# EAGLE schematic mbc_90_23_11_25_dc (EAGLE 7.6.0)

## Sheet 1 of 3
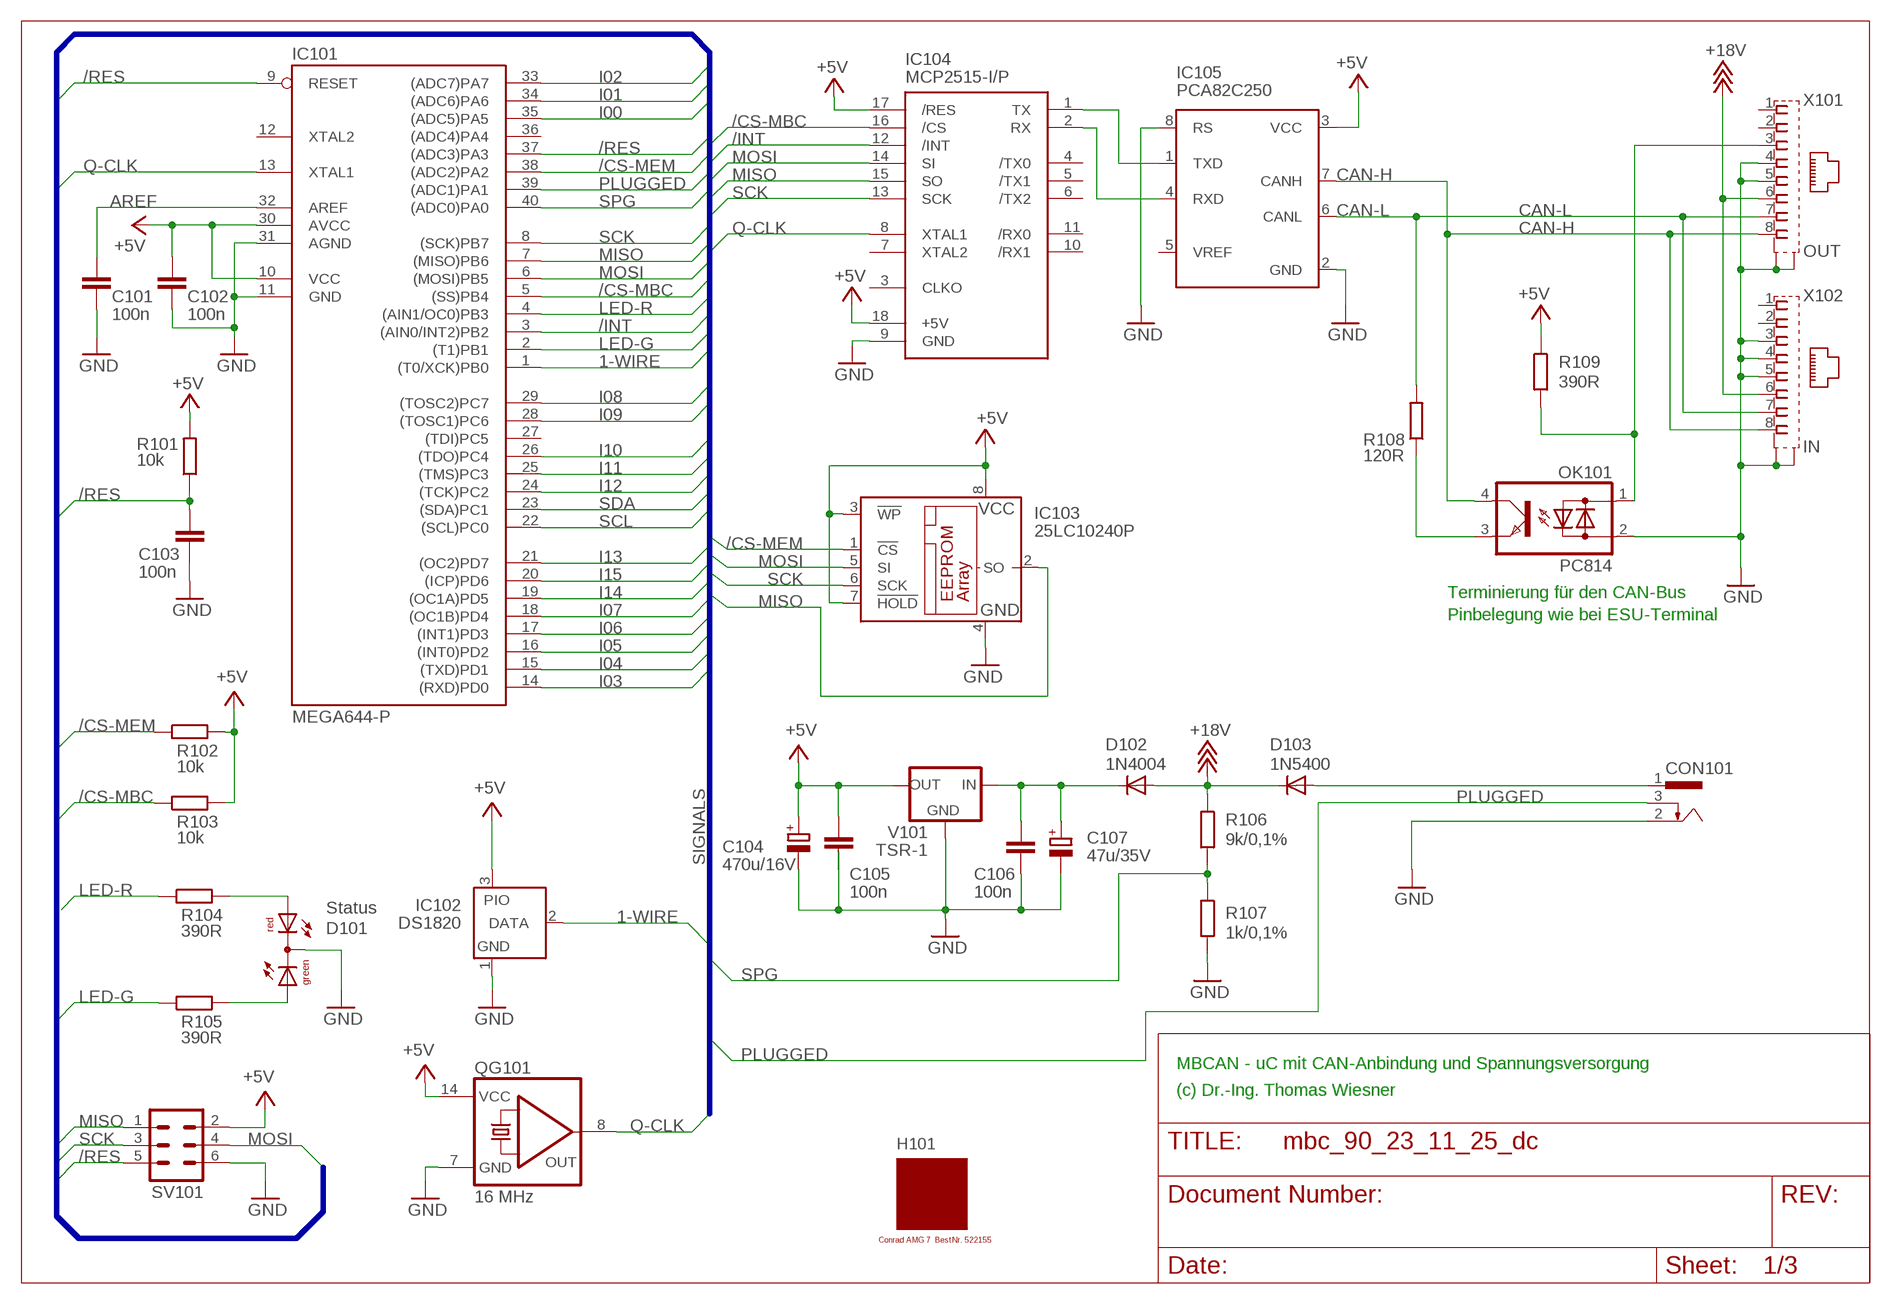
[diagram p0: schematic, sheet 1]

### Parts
C101  100n  C-EU025-025X050  [C025-025X050]
C102  100n  C-EU025-025X050  [C025-025X050]
C103  100n  C-EU025-025X050  [C025-025X050]
C104  470u/16V  CPOL-EUE3.5-8  [E3,5-8]
C105  100n  C-EU025-025X050  [C025-025X050]
C106  100n  C-EU025-025X050  [C025-025X050]
C107  47u/35V  CPOL-EUE2.5-7  [E2,5-7]
CON101  POWER-JACK  [POWER-JACK]
D101  Status  DUOLED5MM  [DUOLED5MM]
D102  1N4004  [DO41-10]
D103  1N5400  [DO201-15]
H101  MODULGEHÄUSE-AMG-7  [MODULGEHÄUSE-1]
IC101  MEGA644-P  MEGA323-P  [DIL40]
IC102  DS1820  DS2405  [TO92-]
IC103  25LC10240P  25LC040P  [DIL8]
IC104  MCP2515-I/P  MCP2510-I/P  [DIL18]
IC105  PCA82C250  [DIL08]
OK101  PC814  [DIL04]
QG101  16 MHz  QG5860  [DIL14S]
R101  10k  R-EU_0207/10  [0207/10]
R102  10k  R-EU_0207/10  [0207/10]
R103  10k  R-EU_0207/10  [0207/10]
R104  390R  R-EU_0207/10  [0207/10]
R105  390R  R-EU_0207/10  [0207/10]
R106  9k/0,1%  R-EU_0207/10  [0207/10]
R107  1k/0,1%  R-EU_0207/10  [0207/10]
R108  120R  R-EU_0207/10  [0207/10]
R109  390R  R-EU_0207/10  [0207/10]
SV101  ML6  [ML6]
V101  TSR-1  [TRACO-TSR-1]
X101  OUT  0446200002  [0446200002]
X102  IN  0446200002  [0446200002]

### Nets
1-WIRE: IC101.1((T0/XCK)PB0) IC102.2(DATA)
+5V: C102.1 C104.+ C105.1 IC101.10(VCC) IC101.30(AVCC) IC102.3(PIO) IC103.3(!WP) IC103.7(!HOLD) IC103.8(VCC) IC104.17(/RES) IC104.18(+5V) IC105.3(VCC) QG101.14(VCC) R101.2 R102.2 R103.2 R109.1 SV101.2 V101.OUT ; also sheet 2
+18V: D102.A D103.C R106.1 X101.6 X102.6
/CS-MBC: IC101.5((SS)PB4) IC104.16(/CS) R103.1
/CS-MEM: IC101.38((ADC2)PA2) IC103.1(!CS) R102.1
/INT: IC101.3((AIN0/INT2)PB2) IC104.12(/INT)
/RES: C103.1 IC101.9(RESET) IC101.37((ADC3)PA3) R101.1 SV101.5
AREF: C101.1 IC101.32(AREF)
CAN-H: IC105.7(CANH) OK101.4(C) X101.8 X102.8
CAN-L: IC105.6(CANL) R108.2 X101.7 X102.7
GND: C101.2 C102.2 C103.2 C104.- C105.2 C106.2 C107.- CON101.2 D101.K(C) IC101.11(GND) IC101.31(AGND) IC102.1(GND) IC103.4(GND) IC104.9(GND) IC105.2(GND) IC105.8(RS) QG101.7(GND) R107.2 SV101.6 V101.GND X101.4 X101.5 X101.S@1(S1) X101.S@2(S2) X102.3 X102.4 X102.5 X102.S@1(S1) X102.S@2(S2) ; also sheet 2
I00: IC101.35((ADC5)PA5) ; also sheet 2
I01: IC101.34((ADC6)PA6) ; also sheet 2
I02: IC101.33((ADC7)PA7) ; also sheet 2
I03: IC101.14((RXD)PD0) ; also sheet 2
I04: IC101.15((TXD)PD1) ; also sheet 2
I05: IC101.16((INT0)PD2) ; also sheet 2
I06: IC101.17((INT1)PD3) ; also sheet 2
I07: IC101.18((OC1B)PD4) ; also sheet 2
I08: IC101.29((TOSC2)PC7) ; also sheet 2
I09: IC101.28((TOSC1)PC6) ; also sheet 2
I10: IC101.26((TDO)PC4) ; also sheet 2
I11: IC101.25((TMS)PC3) ; also sheet 2
I12: IC101.24((TCK)PC2) ; also sheet 2
I13: IC101.21((OC2)PD7) ; also sheet 2
I14: IC101.19((OC1A)PD5) ; also sheet 2
I15: IC101.20((ICP)PD6) ; also sheet 2
LED-G: IC101.2((T1)PB1) R105.1
LED-R: IC101.4((AIN1/OC0)PB3) R104.1
MISO: IC101.7((MISO)PB6) IC103.2(SO) IC104.15(SO) SV101.1
MOSI: IC101.6((MOSI)PB5) IC103.5(SI) IC104.14(SI) SV101.4
N$1: IC104.1(TX) IC105.1(TXD)
N$2: IC104.2(RX) IC105.4(RXD)
N$4: OK101.3(E) R108.1
N$6: C106.1 C107.+ D102.C V101.IN
N$7: OK101.1(AC1) R109.2 X101.3
N$9: D101.AR R104.2
N$13: D101.AG R105.2
PLUGGED: CON101.3 IC101.39((ADC1)PA1)
Q-CLK: IC101.13(XTAL1) IC104.8(XTAL1) QG101.8(OUT)
SCK: IC101.8((SCK)PB7) IC103.6(SCK) IC104.13(SCK) SV101.3
SCL: IC101.22((SCL)PC0) ; also sheet 2
SDA: IC101.23((SDA)PC1) ; also sheet 2
SPG: IC101.40((ADC0)PA0) R106.2 R107.1
V-NETZTEIL1: CON101.1 D103.A
Unconnected: IC101.12(XTAL2) IC101.27((TDI)PC5) IC101.36((ADC4)PA4) IC104.3(CLKO) IC104.4(/TX0) IC104.5(/TX1) IC104.6(/TX2) IC104.7(XTAL2) IC104.10(/RX1) IC104.11(/RX0) IC105.5(VREF) OK101.2(AC2) X101.1 X101.2 X102.1 X102.2

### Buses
SIGNALS

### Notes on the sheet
- Terminierung für den CAN-Bus
- Pinbelegung wie bei ESU-Terminal
- MBCAN - uC mit CAN-Anbindung und Spannungsversorgung
- (c) Dr.-Ing. Thomas Wiesner

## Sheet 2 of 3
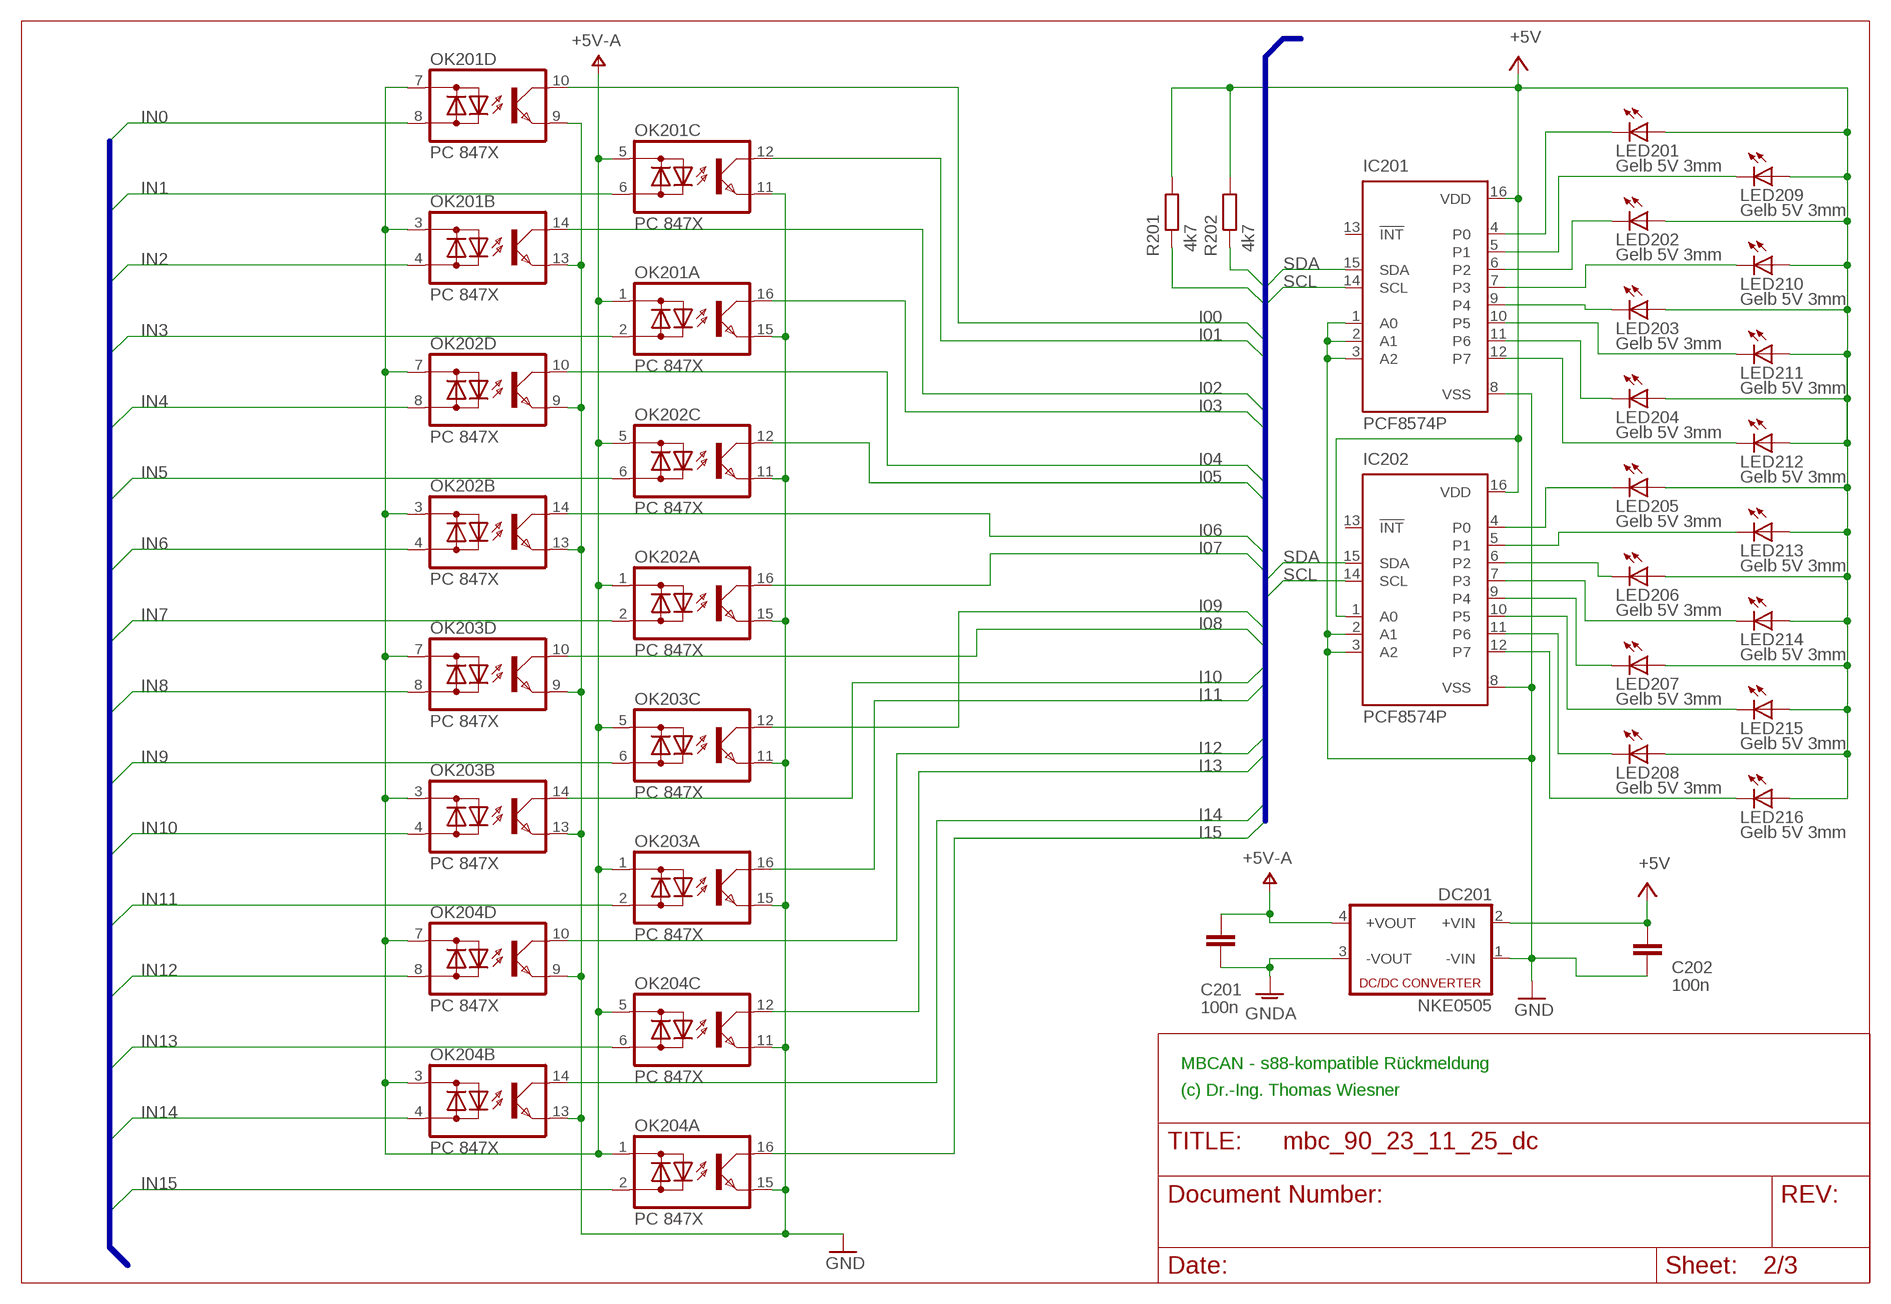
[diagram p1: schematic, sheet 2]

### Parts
C201  100n  C-EU025-025X050  [C025-025X050]
C202  100n  C-EU025-025X050  [C025-025X050]
DC201  NKE0505  NME  [NME]
IC201  PCF8574P  [DIL16]
IC202  PCF8574P  [DIL16]
LED201  Gelb 5V 3mm  LED3MM  [LED3MM]
LED202  Gelb 5V 3mm  LED3MM  [LED3MM]
LED203  Gelb 5V 3mm  LED3MM  [LED3MM]
LED204  Gelb 5V 3mm  LED3MM  [LED3MM]
LED205  Gelb 5V 3mm  LED3MM  [LED3MM]
LED206  Gelb 5V 3mm  LED3MM  [LED3MM]
LED207  Gelb 5V 3mm  LED3MM  [LED3MM]
LED208  Gelb 5V 3mm  LED3MM  [LED3MM]
LED209  Gelb 5V 3mm  LED3MM  [LED3MM]
LED210  Gelb 5V 3mm  LED3MM  [LED3MM]
LED211  Gelb 5V 3mm  LED3MM  [LED3MM]
LED212  Gelb 5V 3mm  LED3MM  [LED3MM]
LED213  Gelb 5V 3mm  LED3MM  [LED3MM]
LED214  Gelb 5V 3mm  LED3MM  [LED3MM]
LED215  Gelb 5V 3mm  LED3MM  [LED3MM]
LED216  Gelb 5V 3mm  LED3MM  [LED3MM]
OK201  PC 847X  TIL196  [DIL16]
OK202  PC 847X  TIL196  [DIL16]
OK203  PC 847X  TIL196  [DIL16]
OK204  PC 847X  TIL196  [DIL16]
R201  4k7  R-EU_0207/10  [0207/10]
R202  4k7  R-EU_0207/10  [0207/10]

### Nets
+5V: C202.1 DC201.2(+VIN) IC201.16(VDD) IC202.1(A0) IC202.16(VDD) LED201.A LED202.A LED203.A LED204.A LED205.A LED206.A LED207.A LED208.A LED209.A LED210.A LED211.A LED212.A LED213.A LED214.A LED215.A LED216.A R201.2 R202.2 ; also sheet 1
GND: C202.2 DC201.1(-VIN) IC201.1(A0) IC201.2(A1) IC201.3(A2) IC201.8(VSS) IC202.2(A1) IC202.3(A2) IC202.8(VSS) OK201.9(D:E) OK201.11(C:E) OK201.13(B:E) OK201.15(A:E) OK202.9(D:E) OK202.11(C:E) OK202.13(B:E) OK202.15(A:E) OK203.9(D:E) OK203.11(C:E) OK203.13(B:E) OK203.15(A:E) OK204.9(D:E) OK204.11(C:E) OK204.13(B:E) OK204.15(A:E) ; also sheet 1
GNDA: C201.2 DC201.3(-VOUT) ; also sheet 3
I00: OK201.10(D:C) ; also sheet 1
I01: OK201.12(C:C) ; also sheet 1
I02: OK201.14(B:C) ; also sheet 1
I03: OK201.16(A:C) ; also sheet 1
I04: OK202.10(D:C) ; also sheet 1
I05: OK202.12(C:C) ; also sheet 1
I06: OK202.14(B:C) ; also sheet 1
I07: OK202.16(A:C) ; also sheet 1
I08: OK203.10(D:C) ; also sheet 1
I09: OK203.12(C:C) ; also sheet 1
I10: OK203.14(B:C) ; also sheet 1
I11: OK203.16(A:C) ; also sheet 1
I12: OK204.10(D:C) ; also sheet 1
I13: OK204.12(C:C) ; also sheet 1
I14: OK204.14(B:C) ; also sheet 1
I15: OK204.16(A:C) ; also sheet 1
IN0: OK201.8(D:AC2) ; also sheet 3
IN1: OK201.6(C:AC2) ; also sheet 3
IN2: OK201.4(B:AC2) ; also sheet 3
IN3: OK201.2(A:AC2) ; also sheet 3
IN4: OK202.8(D:AC2) ; also sheet 3
IN5: OK202.6(C:AC2) ; also sheet 3
IN6: OK202.4(B:AC2) ; also sheet 3
IN7: OK202.2(A:AC2) ; also sheet 3
IN8: OK203.8(D:AC2) ; also sheet 3
IN9: OK203.6(C:AC2) ; also sheet 3
IN10: OK203.4(B:AC2) ; also sheet 3
IN11: OK203.2(A:AC2) ; also sheet 3
IN12: OK204.8(D:AC2) ; also sheet 3
IN13: OK204.6(C:AC2) ; also sheet 3
IN14: OK204.4(B:AC2) ; also sheet 3
IN15: OK204.2(A:AC2) ; also sheet 3
N$15: IC201.9(P4) LED203.K(C)
N$31: IC201.10(P5) LED211.K(C)
N$49: IC202.4(P0) LED205.K(C)
N$50: IC201.4(P0) LED201.K(C)
N$51: IC201.5(P1) LED209.K(C)
N$52: IC201.6(P2) LED202.K(C)
N$53: IC201.7(P3) LED210.K(C)
N$54: IC201.11(P6) LED204.K(C)
N$55: IC201.12(P7) LED212.K(C)
N$56: IC202.9(P4) LED207.K(C)
N$57: IC202.5(P1) LED213.K(C)
N$58: IC202.6(P2) LED206.K(C)
N$59: IC202.7(P3) LED214.K(C)
N$60: IC202.10(P5) LED215.K(C)
N$61: IC202.11(P6) LED208.K(C)
N$62: IC202.12(P7) LED216.K(C)
SCL: IC201.14(SCL) IC202.14(SCL) R201.1 ; also sheet 1
SDA: IC201.15(SDA) IC202.15(SDA) R202.1 ; also sheet 1
V+: C201.1 DC201.4(+VOUT) OK201.1(A:AC1) OK201.3(B:AC1) OK201.5(C:AC1) OK201.7(D:AC1) OK202.1(A:AC1) OK202.3(B:AC1) OK202.5(C:AC1) OK202.7(D:AC1) OK203.1(A:AC1) OK203.3(B:AC1) OK203.5(C:AC1) OK203.7(D:AC1) OK204.1(A:AC1) OK204.3(B:AC1) OK204.5(C:AC1) OK204.7(D:AC1) ; supply symbol labelled +5V-A
Unconnected: IC201.13(!INT) IC202.13(!INT)

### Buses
B$1
B$2

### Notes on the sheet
- MBCAN - s88-kompatible Rückmeldung
- (c) Dr.-Ing. Thomas Wiesner

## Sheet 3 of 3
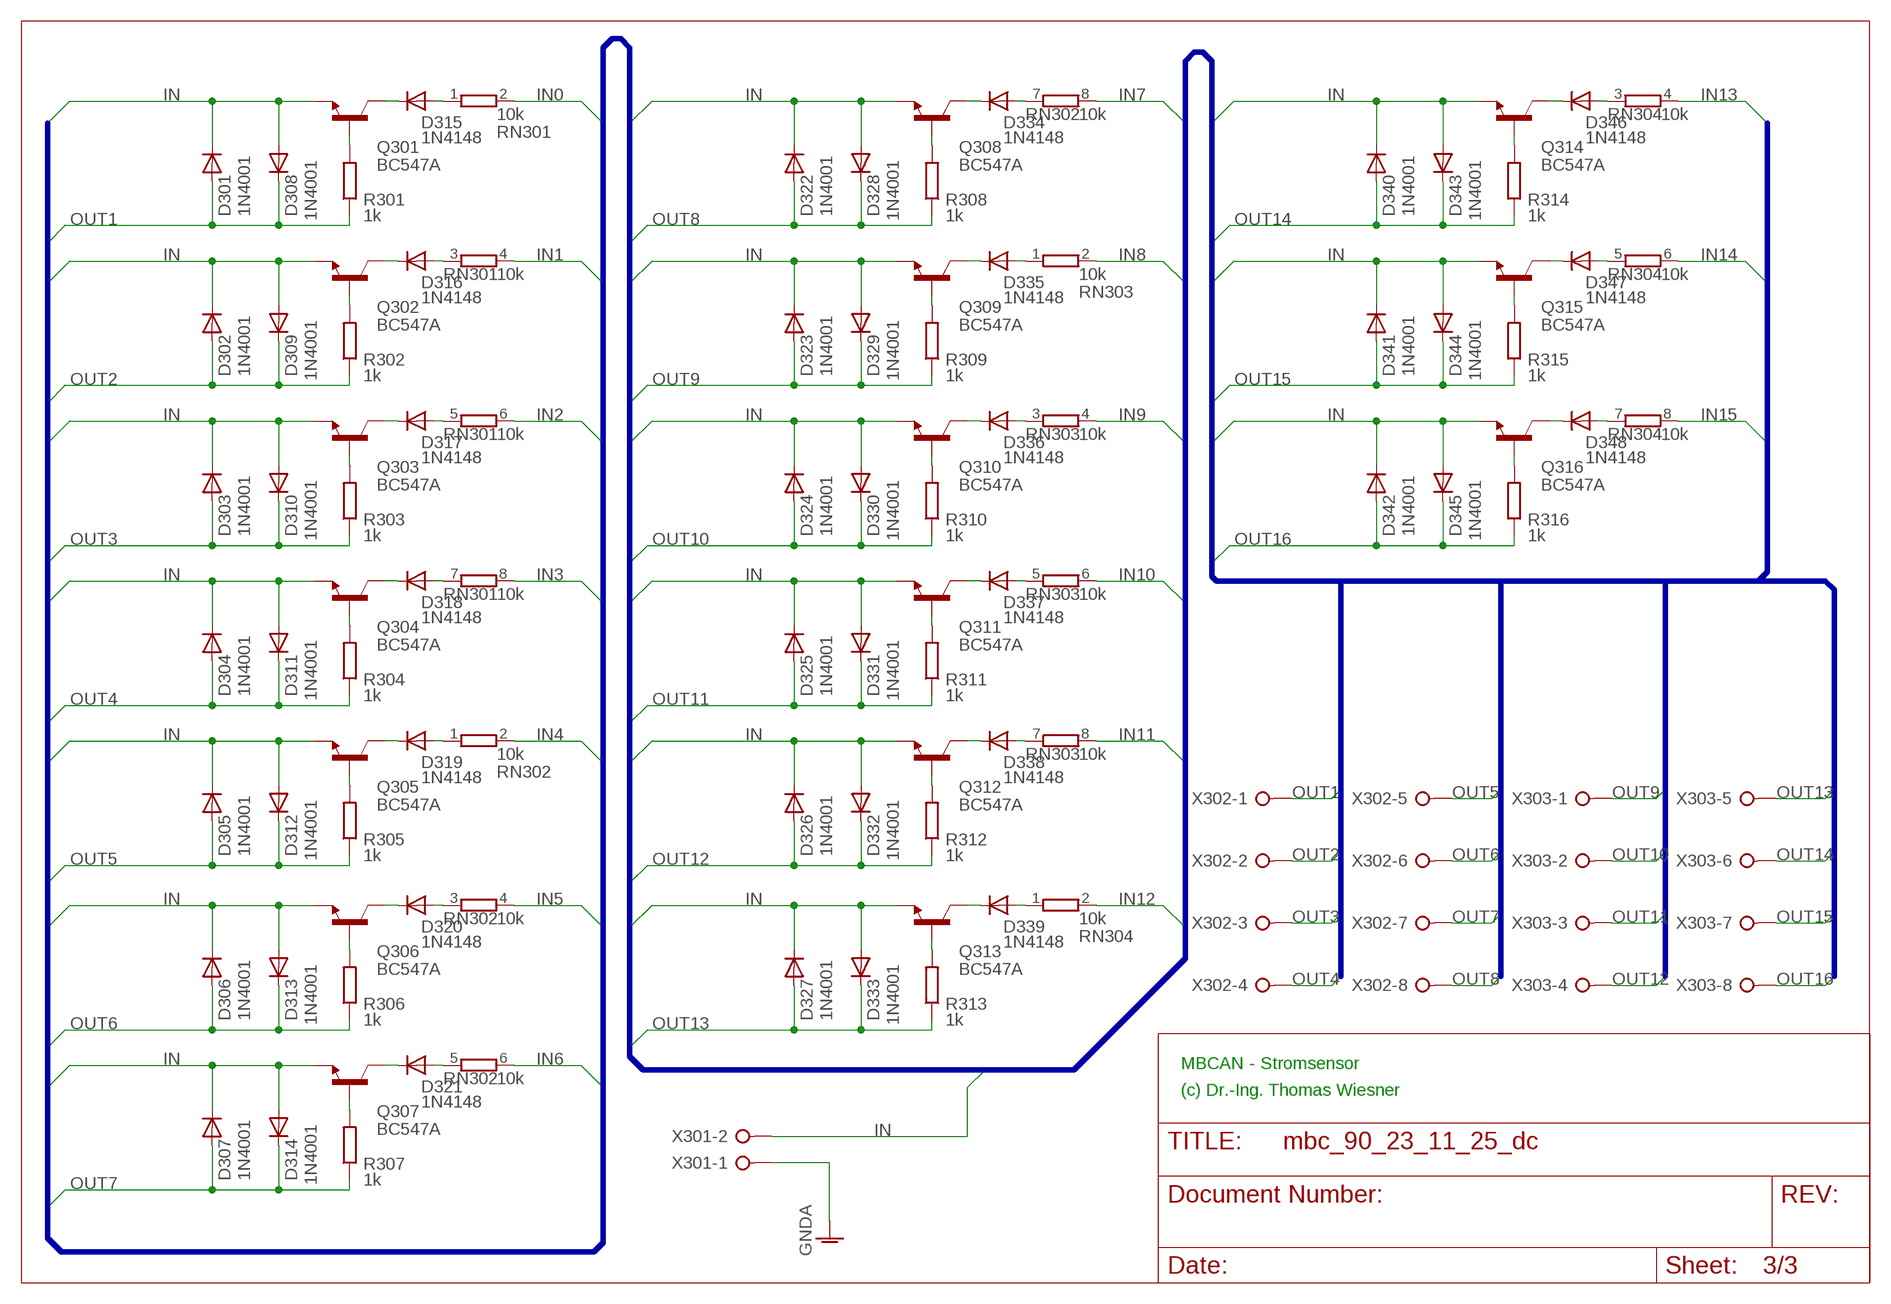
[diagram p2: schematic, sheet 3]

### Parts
D301  1N4001  1N4004  [DO41-10]
D302  1N4001  1N4004  [DO41-10]
D303  1N4001  1N4004  [DO41-10]
D304  1N4001  1N4004  [DO41-10]
D305  1N4001  1N4004  [DO41-10]
D306  1N4001  1N4004  [DO41-10]
D307  1N4001  1N4004  [DO41-10]
D308  1N4001  1N4004  [DO41-10]
D309  1N4001  1N4004  [DO41-10]
D310  1N4001  1N4004  [DO41-10]
D311  1N4001  1N4004  [DO41-10]
D312  1N4001  1N4004  [DO41-10]
D313  1N4001  1N4004  [DO41-10]
D314  1N4001  1N4004  [DO41-10]
D315  1N4148  1N4148DO35-10  [DO35-10]
D316  1N4148  1N4148DO35-10  [DO35-10]
D317  1N4148  1N4148DO35-10  [DO35-10]
D318  1N4148  1N4148DO35-10  [DO35-10]
D319  1N4148  1N4148DO35-10  [DO35-10]
D320  1N4148  1N4148DO35-10  [DO35-10]
D321  1N4148  1N4148DO35-10  [DO35-10]
D322  1N4001  1N4004  [DO41-10]
D323  1N4001  1N4004  [DO41-10]
D324  1N4001  1N4004  [DO41-10]
D325  1N4001  1N4004  [DO41-10]
D326  1N4001  1N4004  [DO41-10]
D327  1N4001  1N4004  [DO41-10]
D328  1N4001  1N4004  [DO41-10]
D329  1N4001  1N4004  [DO41-10]
D330  1N4001  1N4004  [DO41-10]
D331  1N4001  1N4004  [DO41-10]
D332  1N4001  1N4004  [DO41-10]
D333  1N4001  1N4004  [DO41-10]
D334  1N4148  1N4148DO35-10  [DO35-10]
D335  1N4148  1N4148DO35-10  [DO35-10]
D336  1N4148  1N4148DO35-10  [DO35-10]
D337  1N4148  1N4148DO35-10  [DO35-10]
D338  1N4148  1N4148DO35-10  [DO35-10]
D339  1N4148  1N4148DO35-10  [DO35-10]
D340  1N4001  1N4004  [DO41-10]
D341  1N4001  1N4004  [DO41-10]
D342  1N4001  1N4004  [DO41-10]
D343  1N4001  1N4004  [DO41-10]
D344  1N4001  1N4004  [DO41-10]
D345  1N4001  1N4004  [DO41-10]
D346  1N4148  1N4148DO35-10  [DO35-10]
D347  1N4148  1N4148DO35-10  [DO35-10]
D348  1N4148  1N4148DO35-10  [DO35-10]
Q301  BC547A  [TO92]
Q302  BC547A  [TO92]
Q303  BC547A  [TO92]
Q304  BC547A  [TO92]
Q305  BC547A  [TO92]
Q306  BC547A  [TO92]
Q307  BC547A  [TO92]
Q308  BC547A  [TO92]
Q309  BC547A  [TO92]
Q310  BC547A  [TO92]
Q311  BC547A  [TO92]
Q312  BC547A  [TO92]
Q313  BC547A  [TO92]
Q314  BC547A  [TO92]
Q315  BC547A  [TO92]
Q316  BC547A  [TO92]
R301  1k  R-EU_0207/10  [0207/10]
R302  1k  R-EU_0207/10  [0207/10]
R303  1k  R-EU_0207/10  [0207/10]
R304  1k  R-EU_0207/10  [0207/10]
R305  1k  R-EU_0207/10  [0207/10]
R306  1k  R-EU_0207/10  [0207/10]
R307  1k  R-EU_0207/10  [0207/10]
R308  1k  R-EU_0207/10  [0207/10]
R309  1k  R-EU_0207/10  [0207/10]
R310  1k  R-EU_0207/10  [0207/10]
R311  1k  R-EU_0207/10  [0207/10]
R312  1k  R-EU_0207/10  [0207/10]
R313  1k  R-EU_0207/10  [0207/10]
R314  1k  R-EU_0207/10  [0207/10]
R315  1k  R-EU_0207/10  [0207/10]
R316  1k  R-EU_0207/10  [0207/10]
RN301  10k  E4RP  [SIL8]
RN302  10k  E4RP  [SIL8]
RN303  10k  E4RP  [SIL8]
RN304  10k  E4RP  [SIL8]
X301  W237-02P  [W237-132]
X302  W237-08P  [W237-8P]
X303  W237-08P  [W237-8P]

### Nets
GNDA: X301.1 ; also sheet 2
IN: D301.C D302.C D303.C D304.C D305.C D306.C D307.C D308.A D309.A D310.A D311.A D312.A D313.A D314.A D322.C D323.C D324.C D325.C D326.C D327.C D328.A D329.A D330.A D331.A D332.A D333.A D340.C D341.C D342.C D343.A D344.A D345.A Q301.1(E) Q302.1(E) Q303.1(E) Q304.1(E) Q305.1(E) Q306.1(E) Q307.1(E) Q308.1(E) Q309.1(E) Q310.1(E) Q311.1(E) Q312.1(E) Q313.1(E) Q314.1(E) Q315.1(E) Q316.1(E) X301.2
IN0: RN301.2 ; also sheet 2
IN1: RN301.4 ; also sheet 2
IN2: RN301.6 ; also sheet 2
IN3: RN301.8 ; also sheet 2
IN4: RN302.2 ; also sheet 2
IN5: RN302.4 ; also sheet 2
IN6: RN302.6 ; also sheet 2
IN7: RN302.8 ; also sheet 2
IN8: RN303.2 ; also sheet 2
IN9: RN303.4 ; also sheet 2
IN10: RN303.6 ; also sheet 2
IN11: RN303.8 ; also sheet 2
IN12: RN304.2 ; also sheet 2
IN13: RN304.4 ; also sheet 2
IN14: RN304.6 ; also sheet 2
IN15: RN304.8 ; also sheet 2
N$3: Q302.2(B) R302.2
N$5: D316.C Q302.3(C)
N$8: D316.A RN301.3
N$10: Q303.2(B) R303.2
N$11: D317.C Q303.3(C)
N$12: D317.A RN301.5
N$14: Q304.2(B) R304.2
N$16: D318.C Q304.3(C)
N$17: D318.A RN301.7
N$18: Q305.2(B) R305.2
N$19: D319.C Q305.3(C)
N$20: D319.A RN302.1
N$21: Q306.2(B) R306.2
N$22: D320.C Q306.3(C)
N$23: D320.A RN302.3
N$24: Q307.2(B) R307.2
N$25: D321.C Q307.3(C)
N$26: D321.A RN302.5
N$27: Q301.2(B) R301.2
N$28: Q308.2(B) R308.2
N$29: D334.C Q308.3(C)
N$30: D334.A RN302.7
N$32: Q309.2(B) R309.2
N$33: D315.C Q301.3(C)
N$34: D335.C Q309.3(C)
N$35: D335.A RN303.1
N$36: Q310.2(B) R310.2
N$37: D336.C Q310.3(C)
N$38: D315.A RN301.1
N$39: D336.A RN303.3
N$40: Q311.2(B) R311.2
N$41: D337.C Q311.3(C)
N$42: D337.A RN303.5
N$43: Q312.2(B) R312.2
N$44: D338.C Q312.3(C)
N$45: D338.A RN303.7
N$46: Q313.2(B) R313.2
N$47: D339.C Q313.3(C)
N$48: D339.A RN304.1
N$63: Q314.2(B) R314.2
N$64: D346.C Q314.3(C)
N$65: D346.A RN304.3
N$66: Q315.2(B) R315.2
N$67: D347.C Q315.3(C)
N$68: D347.A RN304.5
N$69: Q316.2(B) R316.2
N$70: D348.C Q316.3(C)
N$71: D348.A RN304.7
OUT1: D301.A D308.C R301.1 X302.1
OUT2: D302.A D309.C R302.1 X302.2
OUT3: D303.A D310.C R303.1 X302.3
OUT4: D304.A D311.C R304.1 X302.4
OUT5: D305.A D312.C R305.1 X302.5
OUT6: D306.A D313.C R306.1 X302.6
OUT7: D307.A D314.C R307.1 X302.7
OUT8: D322.A D328.C R308.1 X302.8
OUT9: D323.A D329.C R309.1 X303.1
OUT10: D324.A D330.C R310.1 X303.2
OUT11: D325.A D331.C R311.1 X303.3
OUT12: D326.A D332.C R312.1 X303.4
OUT13: D327.A D333.C R313.1 X303.5
OUT14: D340.A D343.C R314.1 X303.6
OUT15: D341.A D344.C R315.1 X303.7
OUT16: D342.A D345.C R316.1 X303.8

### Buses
B$4

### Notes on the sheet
- MBCAN - Stromsensor
- (c) Dr.-Ing. Thomas Wiesner

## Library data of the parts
C101-C103 C105 C106 C201 C202 = rcl:C-EU: CAPACITOR, European symbol
C104 C107 = rcl:CPOL-EU: POLARIZED CAPACITOR, European symbol
CON101 = mbc:POWER-JACK: Power-Stecker für 2,5 mm Hohlbuchse
D101 = led:DUOLED5MM: DUO LED 2 colors, 5 mm, round
D102 D301-D314 D322-D333 D340-D345 = diode:1N4004: DIODE
D103 = diode:1N5400: DIODE
D315-D321 D334-D339 D346-D348 = diode:1N4148: DIODE
DC201 = dc-dc-converter:NME: DC-DC CONVERTER; MF: C & D TECHNOLOGIES, INC; MPN: NME1205D; OC_FARNELL: 1021466; OC_NEWARK: 98B8198
H101 = mbc:MODULGEHÄUSE-AMG-7: Gehäuse
IC101 = atmel:MEGA323-P: MICROCONTROLLER 32 Kbytes FLASH 2 Kbytes SRAM 1 Kbytes EEPROM USART 8-channel 10 bit ADC Source: avr.lbr; OC_FARNELL: unknown; OC_NEWARK: unknown
IC102 = maxim:DS2405: Addressable Switch DALLAS Semiconductor; MF: DALLAS SEMICONDUCTOR; MPN: DS2405; OC_FARNELL: 1188025; OC_NEWARK: 06F4645
IC103 = microchip:25*: Serial EEPROM 4K/ 8K , SPI bus; MF: MICROCHIP; MPN: 25LC040/P; OC_FARNELL: 9758100; OC_NEWARK: 96K4091
IC104 = mbc:MCP2510: BASIC-CAN 2.0a Controller Stand-alone CAN controller von Microchip
IC105 = micro-philips:PCA82C250: CAN CONTROLLER INTERFACE; OC_FARNELL: 3692358; OC_NEWARK: unknown
IC201 IC202 = micro-philips:PCF8574: I2C-Bus Remote 8-bit I/O expander http://www.semiconductors.philips.com/acrobat_download/datasheets/PCF8574_4.pdf; MPN: PCF8574PN; OC_FARNELL: 204020; OC_NEWARK: 11N8515
LED201-LED216 = led:LED: LED
OK101 = optocoupler:PC814: SHARP OPTO COUPLER; OC_FARNELL: 9707662; OC_NEWARK: unknown
OK201-OK204 = optocoupler:TIL196: TEXAS INSTRUMENTS OPTO COUPLER; MPN: TIL 196; OC_FARNELL: 1683367; OC_NEWARK: 05R6476
Q301-Q316 = transistor-npn:BC547*: NPN Transistor
QG101 = crystal:QG5860: CRYSTAL RESONATOR; OC_FARNELL: unknown; OC_NEWARK: unknown
R101-R109 R201 R202 R301-R316 = resistor:R-EU_: RESISTOR, European symbol
RN301-RN304 = resistor-sil:E4RP: SIL RESISTOR; OC_FARNELL: unknown; OC_NEWARK: unknown
SV101 = con-ml:ML6: HARTING; OC_FARNELL: unknown; OC_NEWARK: unknown
V101 = mbc:TSR-1: Spannungsregler Hersteller: TRACO Typ: TSR-1 5V: TSR 1-2450 Spg: 5V Strom: 1A Reichelt TSR 1-2450
X101 X102 = mbc:0446200002: RJ-45 INVERTED MODULAR JACK ASSEMBLY WITH RJ-11 KEEPOUT FEATURE Source: Data sheet MOLEX 0446200002 BUCHSE, RJ45, GESCHIRMT Source: Farnell; MF: MOLEX; MPN: 0446200002; OC_FARNELL: 9251910
X301 = con-wago-508:W237-02P: WAGO SREW CLAMP; OC_FARNELL: unknown; OC_NEWARK: unknown
X302 X303 = con-wago-508:W237-08P: WAGO SREW CLAMP; OC_FARNELL: unknown; OC_NEWARK: unknown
